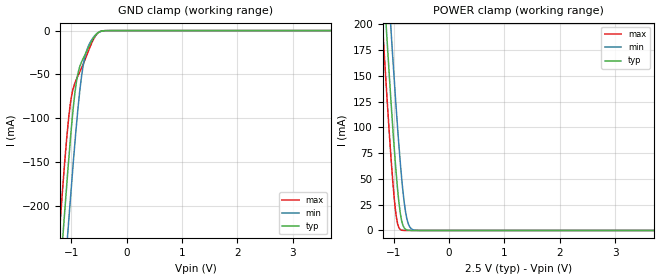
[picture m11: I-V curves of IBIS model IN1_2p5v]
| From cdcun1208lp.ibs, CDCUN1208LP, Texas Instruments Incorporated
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[Model]   IN1_2p5v
Model_type   Input
Vinl = 0.88
Vinh = 1.66
|   typ   min   max
C_comp   9.3930pF   8.2795pF   10.6776pF
[Voltage Range]   2.5   2.375   2.625
[Temperature Range]   27   105   -40
[Power Clamp Reference]   2.5   2.375   2.625
[GND Clamp Reference]   -0   0   0
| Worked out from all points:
|   GND clamp passes 1 mA (typ) near -0.47 V on its own axis
|   POWER clamp passes 1 mA (typ) near -0.78 V on its own axis
[GND Clamp]
|   Voltage   I(typ)   I(min)   I(max)
-2.5V     -1.503A    -1.569A    -1.452A
-1.214V   -289.3mA   -359.7mA   -231.5mA
-1.16V    -242.8mA   -313.4mA   -184.7mA
-1.126V   -213.7mA   -284.6mA   -157mA
-1.055V   -154.7mA   -225.5mA   -105.5mA
-993.8mV  -108.7mA   -175.4mA   -74.5mA
-905.6mV  -58.19mA   -107.8mA   -55.47mA
-844.3mV  -40.94mA   -68.21mA   -46.98mA
-788.2mV  -32.48mA   -41.52mA   -39.06mA
-663.3mV  -16.05mA   -14.21mA   -19.21mA
-473.8mV  -1.055mA   -1.217mA   -912.5uA
4.992V    0A         0A         0A
[POWER Clamp]
|   Voltage   I(typ)   I(min)   I(max)
-2.5V     1.505A     1.572A     1.453A
-1.214V   267.9mA    339.7mA    210.1mA
-1.16V    219.7mA    291.3mA    161.8mA
-1.126V   189.6mA    261.1mA    132.7mA
-1.045V   122.1mA    191.5mA    67.72mA
-993.8mV  82.21mA    149mA      33.05mA
-949.5mV  51.89mA    114.2mA    12.13mA
-879.3mV  16.19mA    64.49mA    877.5uA
-814.8mV  2.923mA    29.08mA    68.76uA
-763.2mV  514.9uA    11.53mA    28.38uA
-638.1mV  18.84uA    497.6uA    26.2uA
4.992V    0A         0A         0A
